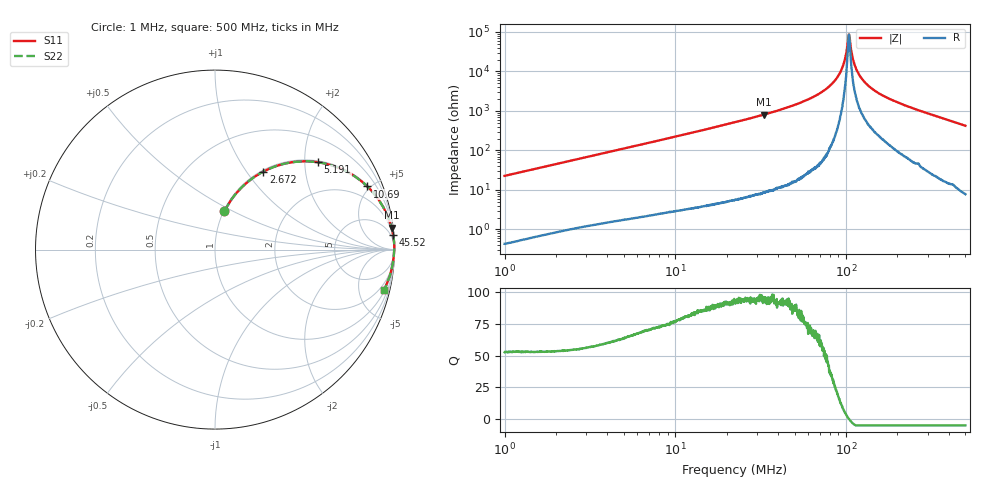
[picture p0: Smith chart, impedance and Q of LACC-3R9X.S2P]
!s-Parameter Generated by FASTRON Sdn. Bhd.
!FASTRON P/N : LACC-3R9X
!Keysight Technologies,E4991B,MY54100416,A.01.15
!Date: Wed Mar 18 09:11:18 2026
!Version  : Rev00 Wed Mar 18 09:11:18 2026
!Data & Calibration Information:
!PortZ  Port1:50+j0  Port2:50+j0
!When reading, reference impedance value at option line is always used.
!Remarks : This data is being provided solely for informational purposes.
!Freq	S11	S21	S12	S22
# Hz S dB R 50
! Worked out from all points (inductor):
!   1601 points, 1 MHz to 500 MHz, reference 50 ohm
!   read as one part in series: L = 3.61 uH near 1.032 MHz
!   highest Q = 95.4 at 33.1 MHz (marker M1), where L = 3.89 uH
!   self-resonance near 103.7 MHz
!   S11 on the Smith chart (normalised r, x): 1 MHz: 1.01, +0.45; 2.672 MHz: 1.02, +1.20; 5.191 MHz: 1.04, +2.32; 10.69 MHz: 1.06, +4.79; 45.52 MHz: 1, +25; 500 MHz: 1.16, -8.43
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1000000  -13.11 76.1  -0.25 -12.8  -0.25 -12.8  -13.11 76.1
2671620  -5.83 58.2  -1.41 -30.7  -1.41 -30.7  -5.83 58.2
2820919  -5.49 56.9  -1.54 -32.1  -1.54 -32.1  -5.49 56.9
5190713  -2.48 40.4  -3.77 -48.8  -3.77 -48.8  -2.48 40.4
7957584  -1.24 29.1  -6.25 -60.1  -6.25 -60.1  -1.24 29.1
1.069011e7  -0.74 22.5  -8.33 -66.7  -8.33 -66.7  -0.74 22.5
2.236068e7  -0.18 10.9  -14.45 -78.5  -14.45 -78.5  -0.18 10.9
3.310225e7  -0.08 7.0  -18.24 -82.4  -18.24 -82.4  -0.08 7.0
4.551764e7  -0.04 4.6  -21.85 -84.7  -21.85 -84.7  -0.04 4.6
6.307767e7  -0.02 2.6  -26.75 -86.5  -26.75 -86.5  -0.02 2.6
7.749595e7  -0.01 1.5  -31.52 -87.2  -31.52 -87.2  -0.01 1.5
8.878078e7  -0.01 0.8  -36.99 -86.3  -36.99 -86.3  -0.01 0.8
9.595246e7  -0.01 0.4  -42.83 -82.6  -42.83 -82.6  -0.01 0.4
9.859709e7  -0.01 0.3  -46.26 -78.2  -46.26 -78.2  -0.01 0.3
1.021047e8  -0.01 0.1  -54.21 -57.0  -54.21 -57.0  -0.01 0.1
1.04107e8  -0.01 -0.0  -58.66 1.9  -58.66 1.9  -0.01 -0.0
1.061486e8  -0.01 -0.1  -53.43 55.1  -53.43 55.1  -0.01 -0.1
1.125168e8  -0.01 -0.4  -43.08 77.1  -43.08 77.1  -0.01 -0.4
1.225542e8  -0.02 -0.8  -36.80 81.5  -36.80 81.5  -0.02 -0.8
1.420459e8  -0.03 -1.6  -31.25 83.0  -31.25 83.0  -0.03 -1.6
1.77937e8  -0.04 -2.8  -26.30 83.3  -26.30 83.3  -0.04 -2.8
5e8  -0.27 -13.3  -12.77 75.6  -12.77 75.6  -0.27 -13.3
